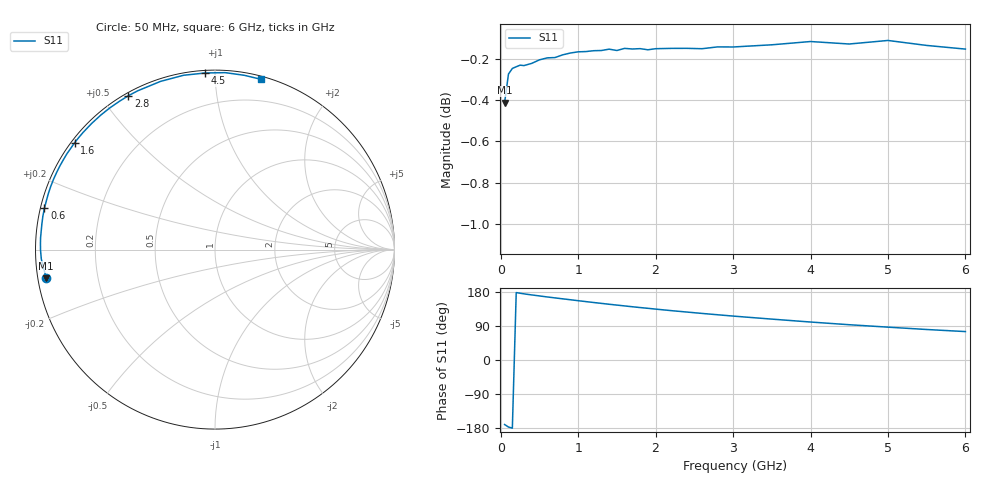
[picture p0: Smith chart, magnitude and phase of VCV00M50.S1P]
! Infineon Technologies  Discrete & RF Semiconductors
! BBY 56-03
! Si Tuning Diode in SOD323
! VR =
! S-Parameters:  June  1999
# GHz  S  MA  R  50
!  f  S11
! GHz  MAG  ANG
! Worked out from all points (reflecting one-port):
!   34 points, 50 MHz to 6 GHz, reference 50 ohm
!   lowest |S11| = -0.4 dB at 50 MHz (marker M1), VSWR 42.24, Z = 1.19 - j4.24 ohm
!   phase of S11 starts at -170 deg and turns -115 deg over the sweep
!   S11 on the Smith chart (normalised r, x): 50 MHz: 0.02, -0.08; 600 MHz: 0.01, +0.12; 1.6 GHz: 0.01, +0.34; 2.8 GHz: 0.01, +0.58; 4.5 GHz: 0.01, +0.95; 6 GHz: 0.02, +1.30
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0.05  0.9537 -170.3
0.1  0.9691 -176.9
0.15  0.9722 -179.9
0.2  0.9731 177.9
0.3  0.9737 174.6
0.4  0.9749 171.7
0.5  0.9769 169.1
0.6  0.9779 166.4
0.8  0.9796 161.4
0.9  0.9806 159.0
1  0.9813 156.5
1.2  0.9819 151.7
1.4  0.9827 147.1
1.6  0.9831 142.7
1.7  0.9828 140.5
1.8  0.983 138.4
2  0.983 134.3
2.2  0.9831 130.3
2.4  0.9832 126.6
2.6  0.983 122.9
2.8  0.984 119.4
3  0.9839 115.9
3.5  0.9851 107.9
4  0.9869 100.2
4.5  0.9856 93.1
5  0.9875 86.7
5.5  0.9848 80.5
6  0.9828 75.0
